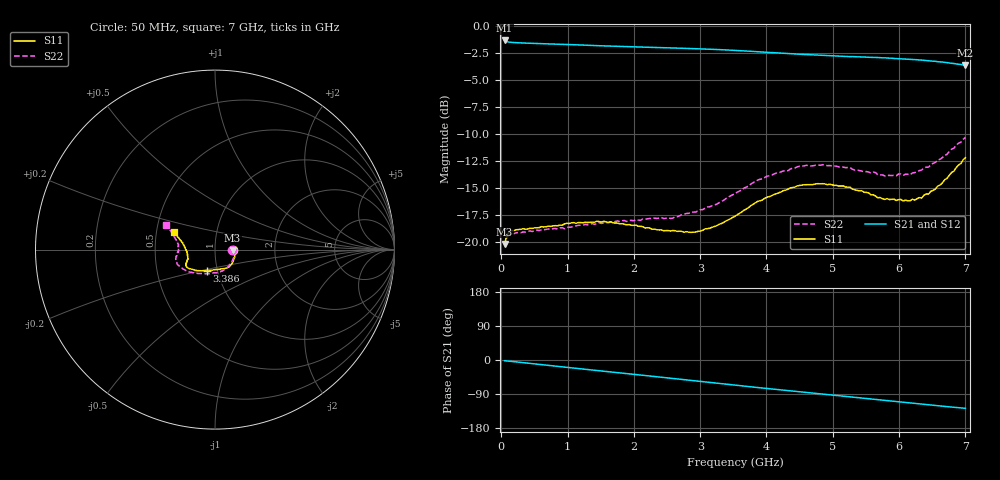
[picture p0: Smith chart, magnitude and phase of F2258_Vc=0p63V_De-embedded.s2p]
! Integrated Device Technology
! Corporate Headquarters
! 6024 Silver Creek Valley Road
! San Jose, CA 95138  USA
! Phone:  1-408-284-8200
! Toll Free:  1-800-223-1366
! Webpage:  http://www.idt.com/
! Timing and RF Division
! 515 Groton Road, Suite 102
! Westford, MA 01886-6024
! Device:  F2258
! Description: Voltage Variable RF Attenuator
! Frequency:  50.0 -  6000.00 MHz
! Package:  3x3 mm Thin QFN Plastic Package: 16 pin
! Ports:  2 RF, 2 DC
!  Pin  1  = NC
!  Pin  2  = NC
!  Pin  3  = RF2  = Port 2
!  Pin  4  = GND
!  Pin  5  = Vdd
!  Pin  6  = NC
!  Pin  7  = VCTRL
!  Pin  8  = NC
!  Pin  9  = GND
!  Pin 10  = RF1  = Port 1
!  Pin 11  = NC
!  Pin 12  = NC
!  Pin 13  = NC
!  Pin 14  = NC
!  Pin 15  = NC
!  Pin 16  = NC
! Vcntrl:  0.630 Volts
! Vdd:  +3.300 Volts
! Current:  1.113 mA
! Data:  The device was measured on a the F2258 evaluation board which has
!  individual transmission lines to the RF pins.  Data was collected
!  using a calibrated network analyzer.  The evaluation board was
!  de-embedded using a TRL calibration technique.
!  The reference plane is the edge of the package pin.
! Misc:  SN 10
!  Action Tracker AT0285
! Date Measured:  2014-12-10
! Date:  2016-01-13  MJV
! Note:
!  Integrated Device Technology supplies this data as a sample of measured
!  data at the package pin for this product.  Your particular data for this
!  product may vary.
!  Data was taken at 25 degrees C.
!  Integrated Device Technology reserves the right to change this data at anytime.
!Freq_(GHz)  S11M_(dB)  S11P_(deg)  S21M_(dB)  S21P_(deg)  S12M_(dB)  S12P_(deg)  S22M_(dB)  S22P_(deg)
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# GHz S dB R 50
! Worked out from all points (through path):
!   201 points, 50 MHz to 7 GHz, reference 50 ohm
!   highest |S21| = -1.36 dB at 50 MHz (marker M1); lowest = -3.7 dB at 7 GHz (marker M2)
!   group delay of S21, straight-line fit = 50.5 ps
!   lowest |S11| = -20.2 dB at 50 MHz (marker M3), VSWR 1.22, Z = 60.8 - j0.493 ohm
!   |S11| at or under -10 dB: start of sweep to end of sweep
!   |S22| runs from -20.4 to -10.3 dB; largest |S21 - S12| = 0.0011
!   S11 on the Smith chart (normalised r, x): 50 MHz: 1.22, -0.01; 3.386 GHz: 0.89, -0.21; 7 GHz: 0.62, +0.13
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0.05  -20.19 -2.4  -1.36 -2.0  -1.36 -2.0  -20.38 -2.7
0.08475  -19.35 -3.9  -1.47 -2.5  -1.47 -2.5  -19.56 -4.3
0.15425  -18.95 -6.1  -1.54 -3.7  -1.54 -3.7  -19.23 -7.5
0.71025  -18.54 -26.3  -1.68 -14.2  -1.68 -14.2  -18.79 -31.6
0.9535  -18.32 -35.7  -1.72 -18.8  -1.73 -18.8  -18.78 -43.2
1.2315  -18.22 -43.6  -1.79 -23.9  -1.79 -23.9  -18.44 -53.5
1.6485  -18.14 -53.5  -1.88 -31.5  -1.88 -31.5  -18.15 -66.5
2.37825  -18.89 -69.9  -2.02 -44.8  -2.02 -44.8  -17.79 -85.8
2.552  -18.99 -75.0  -2.05 -48.0  -2.05 -48.0  -17.83 -91.1
2.93425  -19.07 -90.0  -2.13 -55.1  -2.13 -55.1  -17.23 -104.8
3.386  -18.06 -111.1  -2.24 -63.7  -2.24 -63.6  -15.99 -123.2
3.525  -17.61 -117.0  -2.28 -66.3  -2.29 -66.3  -15.52 -128.3
4.0115  -15.85 -135.0  -2.46 -75.3  -2.47 -75.3  -13.91 -145.0
4.46325  -14.82 -145.4  -2.63 -83.5  -2.63 -83.5  -13.05 -156.9
4.7065  -14.68 -148.8  -2.70 -87.7  -2.70 -87.7  -12.95 -161.5
5.2625  -14.94 -155.0  -2.86 -97.4  -2.86 -97.4  -13.12 -170.3
5.6795  -15.91 -160.1  -2.94 -104.6  -2.94 -104.6  -13.79 -176.3
5.85325  -16.07 -164.1  -3.00 -107.7  -3.00 -107.7  -13.84 179.0
6.166  -16.19 -172.4  -3.10 -113.3  -3.10 -113.2  -13.79 172.5
6.33975  -15.94 -179.9  -3.18 -116.4  -3.18 -116.4  -13.34 167.9
6.61775  -14.74 168.2  -3.34 -121.2  -3.34 -121.2  -12.35 161.1
7  -12.20 157.0  -3.66 -127.4  -3.66 -127.4  -10.32 153.1
